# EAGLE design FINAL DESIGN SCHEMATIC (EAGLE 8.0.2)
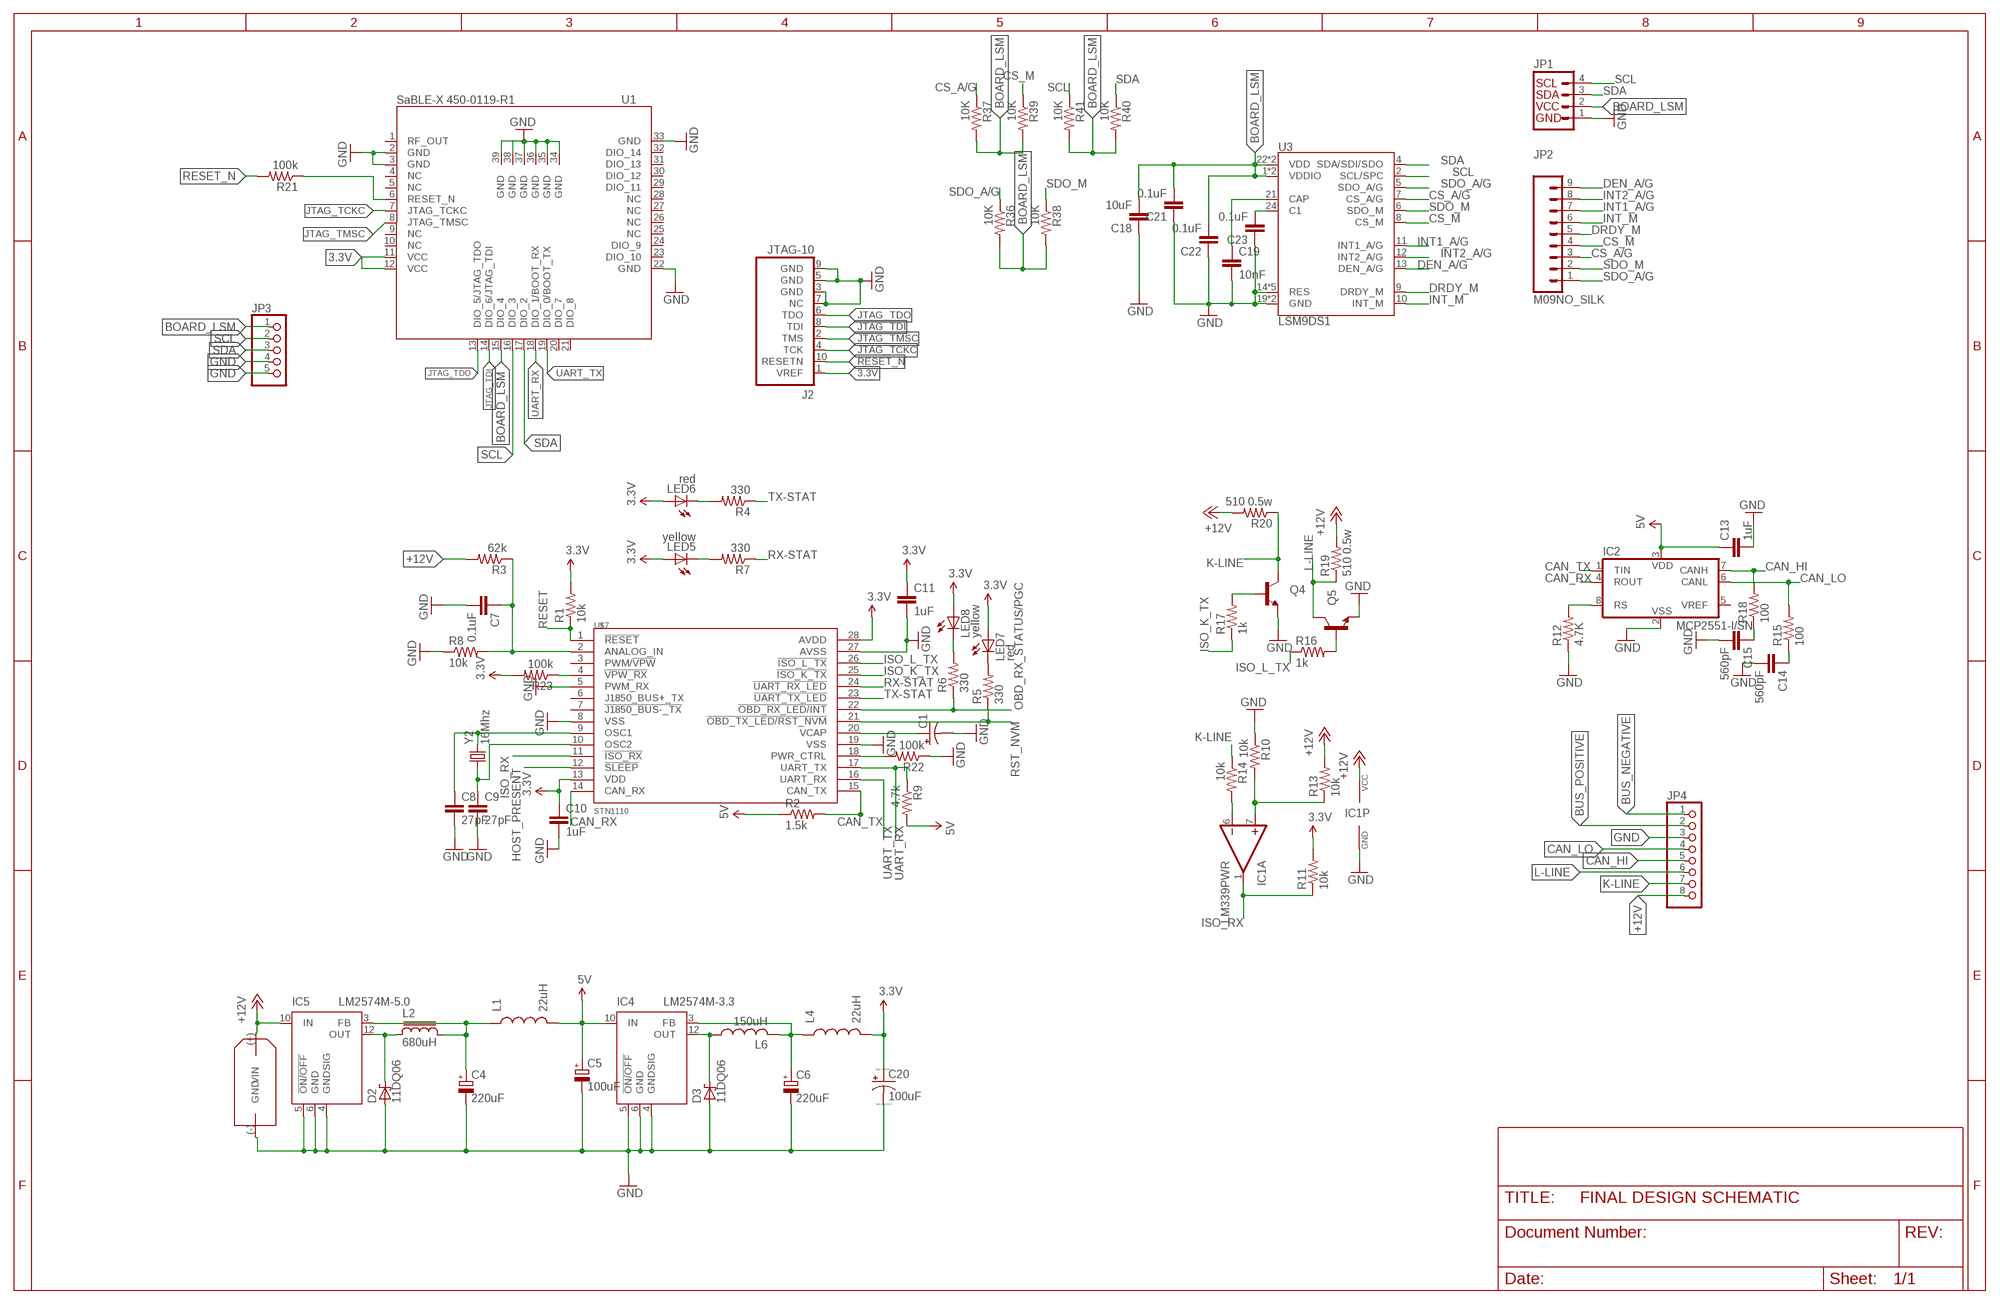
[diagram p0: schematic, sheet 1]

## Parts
C1  CAP_POL1206  [EIA3216]
C4  220uF  CPOL-EUUD-8X10  [UD-8X10_NICHICON]
C5  100uF  CPOL-EUUD-8X10  [UD-8X10_NICHICON]
C6  220uF  CPOL-EUUD-6,3X7,7  [UD-6,3X7,7_NICHICON]
C7  0.1uF  CAP0402-CAP  [0402-CAP]
C8  27pF  CAP0402-CAP  [0402-CAP]
C9  27pF  CAP0402-CAP  [0402-CAP]
C10  1uF  CAP0402-CAP  [0402-CAP]
C11  1uF  CAP0402-CAP  [0402-CAP]
C13  1uF  CAP0402-CAP  [0402-CAP]
C14  560pF  CAP0402-CAP  [0402-CAP]
C15  560pF  CAP0402-CAP  [0402-CAP]
C18  10uF  10UF-6.3V-20%(0603)  [0603-CAP]
C19  10nF  10UF-6.3V-20%(0603)  [0603-CAP]
C20  100uF  CPOL-US139CLL-3R  [139CLL-3R]
C21  0.1uF  0.1UF-25V(+80/-20%)(0603)  [0603-CAP]
C22  0.1uF  0.1UF-25V(+80/-20%)(0603)  [0603-CAP]
C23  0.1uF  0.1UF-25V(+80/-20%)(0603)  [0603-CAP]
CIN1  22uF  MAL214699801E3  [146CTI]
D2  11DQ06  1N5817-T  [DO41-7.6]
D3  11DQ06  1N5817-T  [DO41-7.6]
IC1  LM339PWR  [TSSOP-14]
IC2  MCP2551-I/SN  [SO-8]
IC4  LM2574M-3.3  [SO14W]
IC5  LM2574M-5.0  [SO14W]
J2  JTAG-10  [JTAG-10]
JP1  I2C_STANDARD_NO_SILK  [1X04_NO_SILK]
JP2  M09NO_SILK  [1X09_NO_SILK]
JP3  PINHD-1X5  [1X05]
JP4  PINHD-1X8  [1X08]
L1  22uH  INDUCTOR1210  [1210]
L2  680uH  SDR1006  [SDR1006]
L4  22uH  INDUCTOR1210  [1210]
L6  150uH  L-USL1812  [L1812]
LED5  yellow  LED0603  [LED-0603]
LED6  red  LED0603  [LED-0603]
LED7  red  LED0603  [LED-0603]
LED8  yellow  LED0603  [LED-0603]
Q4  TRANSISTOR_NPNSOT23-3  [SOT23-3]
Q5  TRANSISTOR_NPNSOT23-3  [SOT23-3]
R1  10k  RESISTOR0402-RES  [0402-RES]
R2  1.5k  RESISTOR0402-RES  [0402-RES]
R3  62k  RESISTOR0402-RES  [0402-RES]
R4  330  RESISTOR0402-RES  [0402-RES]
R5  330  RESISTOR0402-RES  [0402-RES]
R6  330  RESISTOR0402-RES  [0402-RES]
R7  330  RESISTOR0402-RES  [0402-RES]
R8  10k  RESISTOR0402-RES  [0402-RES]
R9  4.7k  RESISTOR0402-RES  [0402-RES]
R10  10k  RESISTOR0402-RES  [0402-RES]
R11  10k  RESISTOR0402-RES  [0402-RES]
R12  4.7K  RESISTOR0402-RES  [0402-RES]
R13  10k  RESISTOR0402-RES  [0402-RES]
R14  10k  RESISTOR0402-RES  [0402-RES]
R15  100  RESISTOR0402-RES  [0402-RES]
R16  1k  RESISTOR0402-RES  [0402-RES]
R17  1k  RESISTOR0402-RES  [0402-RES]
R18  100  RESISTOR0402-RES  [0402-RES]
R19  510 0.5w  RESISTOR2010  [R2010]
R20  510 0.5w  RESISTOR2010  [R2010]
R21  100k  RESISTOR0402-RES  [0402-RES]
R22  100k  RESISTOR0402-RES  [0402-RES]
R23  100k  RESISTOR0402-RES  [0402-RES]
R36  10K  10KOHM-1/10W-1%(0603)0603  [0603-RES]
R37  10K  10KOHM-1/10W-1%(0603)0603  [0603-RES]
R38  10K  10KOHM-1/10W-1%(0603)0603  [0603-RES]
R39  10K  10KOHM-1/10W-1%(0603)0603  [0603-RES]
R40  10K  10KOHM-1/10W-1%(0603)0603  [0603-RES]
R41  10K  10KOHM-1/10W-1%(0603)0603  [0603-RES]
U1  SABLEXTRACE-ANTENNA  [SABLEX_450-0119]
U3  LSM9DS1  [LGA24-8X4]
U$7  STN1110  [SO-28W]
Y2  16Mhz  CRYSTAL5X3  [CRYSTAL-SMD-5X3]

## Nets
3.3V [power]: C10.1 C11.1 C20.+ J2.1(VREF) L4.2 LED5.A LED6.A LED7.A LED8.A R1.2 R11.2 R23.2 U1.11(VCC) U1.12(VCC) U$7.13(VDD) U$7.28(AVDD)
5V [power]: C5.+ C13.1 IC2.3(VDD) IC4.10(IN) L1.2 R2.1 R9.2
+12V [power]: CIN1.(+)(VIN) IC1.3(P:VCC) IC5.10(IN) JP4.8 R3.2 R13.2 R19.2 R20.2
BOARD_LSM: C18.2 C21.2 C22.2 JP1.2 JP3.1 R36.2 R37.2 R38.2 R39.2 R40.2 R41.2 U1.15(DIO_4) U3.1(VDDIO) U3.3(VDDIO) U3.22(VDD) U3.23(VDD)
BUS_NEGATIVE: JP4.1
BUS_POSITIVE: JP4.2
CAN_HI: IC2.7(CANH) JP4.5 R18.2
CAN_LO: IC2.6(CANL) JP4.4 R15.2
CAN_RX: IC2.4(ROUT) U$7.14(CAN_RX)
CAN_TX: IC2.1(TIN) R2.2 U$7.15(CAN_TX)
CS_A/G: JP2.3 R37.1 U3.7(CS_A/G)
CS_M: JP2.4 R39.1 U3.8(CS_M)
DEN_A/G: JP2.9 U3.13(DEN_A/G)
DRDY_M: JP2.5 U3.9(DRDY_M)
GND [power]: C1.C(-) C4.- C5.- C6.- C7.2 C8.2 C9.2 C10.2 C11.2 C13.2 C14.2 C15.2 C18.1 C19.2 C20.- C21.1 C22.1 C23.1 CIN1.(-)(GND) D2.A D3.A IC1.12(P:GND) IC2.2(VSS) IC4.4(GNDSIG) IC4.5(!ON/OFF) IC4.6(GND) IC5.4(GNDSIG) IC5.5(!ON/OFF) IC5.6(GND) J2.3(GND) J2.5(GND) J2.7(NC) J2.9(GND) JP1.1 JP3.4 JP3.5 JP4.3 Q4.2(E) Q5.2(E) R8.1 R10.1 R12.1 R22.1 U1.2(GND) U1.3(GND) U1.22(GND) U1.33(GND) U1.34(GND) U1.35(GND) U1.36(GND) U1.37(GND) U1.38(GND) U1.39(GND) U3.14(RES) U3.15(RES) U3.16(RES) U3.17(RES) U3.18(RES) U3.19(GND) U3.20(GND) U$7.5(PWM_RX) U$7.8(VSS) U$7.19(VSS) U$7.27(AVSS)
HOST_PRESENT: U$7.12(!SLEEP)
INT1_A/G: JP2.7 U3.11(INT1_A/G)
INT2_A/G: JP2.8 U3.12(INT2_A/G)
INT_M: JP2.6 U3.10(INT_M)
ISO_K_TX: R17.1 U$7.25(!ISO_K_TX)
ISO_L_TX: R16.1 U$7.26(!ISO_L_TX)
ISO_RX: IC1.1(A:OUT) R11.1 U$7.11(!ISO_RX)
JTAG_TCKC: J2.4(TCK) U1.7(JTAG_TCKC)
JTAG_TDI: J2.8(TDI) U1.14(DIO_6/JTAG_TDI)
JTAG_TDO: J2.6(TDO) U1.13(DIO_5/JTAG_TDO)
JTAG_TMSC: J2.2(TMS) U1.8(JTAG_TMSC)
K-LINE: JP4.7 Q4.3(C) R14.1 R20.1
L-LINE: JP4.6 Q5.3(C) R19.1
N$1 [power]: C8.1 U$7.9(OSC1) Y2.3
N$2: R23.1 U$7.4(!VPW_RX)
N$3 [power]: D3.C IC4.12(OUT) L6.1
N$4 [power]: C4.+ IC5.3(FB) L1.1 L2.2
N$5 [power]: D2.C IC5.12(OUT) L2.1
N$6: R21.1 U1.6(RESET_N)
N$7: R22.2 U$7.18(PWR_CTRL)
N$8 [power]: C6.+ IC4.3(FB) L4.1 L6.2
N$11: LED7.C R5.2
N$15: C19.1 U3.21(CAP)
N$16: C23.2 U3.24(C1)
N$29: Q4.1(B) R17.2
N$34: IC2.8(RS) R12.2
N$35: IC1.7(A:+IN) R10.2 R13.1
N$40: C15.1 R18.1
N$41: C14.1 R15.1
N$42: IC1.6(A:-IN) R14.2
N$43: Q5.1(B) R16.2
N$44: C9.1 U$7.10(OSC2) Y2.1
N$47: C7.1 R3.1 R8.2 U$7.2(ANALOG_IN)
N$48: LED5.C R7.2
N$49: C1.A(+) U$7.20(VCAP)
N$50: LED8.C R6.2
N$51: LED6.C R4.2
OBD_RX_STATUS/PGC: R6.1 U$7.22(!OBD_RX_LED/INT)
RESET: R1.1 U$7.1(!RESET)
RESET_N: J2.10(RESETN) R21.2
RST_NVM: R5.1 U$7.21(!OBD_TX_LED/RST_NVM)
RX-STAT: R7.1 U$7.24(!UART_RX_LED)
SCL: JP1.4 JP3.2 R41.1 U1.16(DIO_3) U3.2(SCL/SPC)
SDA: JP1.3 JP3.3 R40.1 U1.17(DIO_2) U3.4(SDA/SDI/SDO)
SDO_A/G: JP2.1 R36.1 U3.5(SDO_A/G)
SDO_M: JP2.2 R38.1 U3.6(SDO_M)
TX-STAT: R4.1 U$7.23(!UART_TX_LED)
UART_RX: R9.1 U1.18(DIO_1/BOOT_RX) U$7.17(UART_TX)
UART_TX: U1.19(DIO_0/BOOT_TX) U$7.16(UART_RX)
Unconnected: IC1.2(B:OUT) IC1.4(B:-IN) IC1.5(B:+IN) IC1.8(C:-IN) IC1.9(C:+IN) IC1.10(D:-IN) IC1.11(D:+IN) IC1.13(D:OUT) IC1.14(C:OUT) IC2.5(VREF) U1.1(RF_OUT) U1.4(NC) U1.5(NC) U1.9(NC) U1.10(NC) U1.20(DIO_7) U1.21(DIO_8) U1.23(DIO_10) U1.24(DIO_9) U1.25(NC) U1.26(NC) U1.27(NC) U1.28(NC) U1.29(DIO_11) U1.30(DIO_12) U1.31(DIO_13) U1.32(DIO_14) U$7.3(PWM/!VPW) U$7.6(J1850_BUS+_TX) U$7.7(!J1850_BUS-_TX)

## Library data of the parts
C1 = OBD-II-UART-v13:CAP_POL: Capacitor Polarized
C4-C6 = FINAL DESIGN SCHEMATIC (Updated):CPOL-EU: POLARIZED CAPACITOR, European symbol
C7-C11 C13 = OBD-II-UART-v13:CAP: Capacitor; MPN: 2450L/C402D; OC_NEWARK: 55T4197
C14 C15 = OBD-II-UART-v13:CAP: Capacitor; OC_NEWARK: unknown
C18 = SparkFun-LSM9DS1-Breakout:10UF-6.3V-20%(0603): CAP-11015; OC_NEWARK: unknown; PROD_ID: CAP-11015
C19 = SparkFun-LSM9DS1-Breakout:10UF-6.3V-20%(0603): CAP-11015; OC_NEWARK: unknown; PROD_ID: CAP-11015; VALUE: 10uF
C20 = resistor:CPOL-US: POLARIZED CAPACITOR, American symbol
C21-C23 = SparkFun-LSM9DS1-Breakout:0.1UF-25V(+80/-20%)(0603): CAP-00810; OC_NEWARK: unknown; PROD_ID: CAP-00810
CIN1 = FINAL DESIGN SCHEMATIC (Updated):MAL214699801E3
D2 D3 = diode:1N581*: 1.0A SCHOTTKY BARRIER RECTIFIER
IC1 = OBD-II-UART-v13:LM339PWR: Quad Differential Comparators Based on information from the SLCS006N datasheet from TI (www.ti.com). Change Log DateAuthorChange July 16, 2008nick@scantool.netDevice created.; DESC: IC, Quad Comparator; MANUF: Texas Instruments; OC_NEWARK: unknown; PARTNUM: LM339PWR; SUPPLIER: Digikey:296-6607-1-ND; VALSTAT: PARTNUM
IC2 = OBD-II-UART-v13:MCP2551: CAN Driver Based on information from the MPC2551 datasheet from Microchip. http://www.microchip.com/ Change Log DateAuthorChange November 12, 2008joe@scantool.netRenamed "TXD" to "TIN" and "RXD" to "ROUT" Fixed mislabeled pins "CANH" and CANL"; DESC: IC, CAN Transceiver; MANUF: Microchip Technology; OC_NEWARK: unknown; PARTNUM: MCP2551-I/SN; SUPPLIER: Digikey:MCP2551-I/SN-ND; VALSTAT: PARTNUM
IC4 IC5 = linear:LM2574?-*: SIMPLE SWITCHER 0.5A Step-Down Voltage Regulator Source: http://cache.national.com/ds/LM/LM2574.pdf
J2 = luminary-arm:JTAG-10: JTAG 10-Pin Programming/Debug Connector
JP1 = SparkFun-LSM9DS1-Breakout:I2C_STANDARD: SparkFun has standardized on a pinout for all I2C based sensor breakouts. This pinout allows I2C boards to be plugged directly into the headers on Arduino Uno compatible boards, and to be daisy chained easily.; OC_NEWARK: unknown
JP2 = SparkFun-LSM9DS1-Breakout:M09: Header 9 Standard 9-pin 0.1" header. Use with straight break away headers (SKU : PRT-00116), right angle break away headers (PRT-00553), swiss pins (PRT-00743), machine pins (PRT-00117), and female headers (PRT-00115).; OC_NEWARK: unknown
JP3 = pinhead:PINHD-1X5: PIN HEADER
JP4 = pinhead:PINHD-1X8: PIN HEADER
L1 L4 = SparkFun-Passives:INDUCTOR: Inductors
L2 = inductor-bourns:SDR1006: POWER INDUCTOR
L6 = resistor:L-US: INDUCTOR, American symbol
LED5-LED8 = OBD-II-UART-v13:LED: LEDs; OC_NEWARK: unknown
Q4 Q5 = OBD-II-UART-v13:TRANSISTOR_NPN: Transistor NPN BJT configuration in SOT23 package. MMBT2222 is the common NPN we use. Double check BCE configuration again layout.; OC_NEWARK: unknown
R1-R23 = OBD-II-UART-v13:RESISTOR: Resistor; OC_NEWARK: unknown
R36-R41 = SparkFun-LSM9DS1-Breakout:10KOHM-1/10W-1%(0603): RES-00824; OC_NEWARK: unknown; PROD_ID: RES-00824
U1 = sablex:SABLEX: LSR SaBLE-x 450-0119-R1 Technical Specifications: Product Description: Bluetooth Low Energy Wireless Module VCC: 1.8v - 3.8v Operating Temperature: -40c - 85c Weight: 0.75g +/- 0.05f; OC_NEWARK: unknown
U3 = SparkFun-LSM9DS1-Breakout:LSM9DS1: LSM9DS1 3D accelerometer, gyroscope & magnetometer The LSM9DS1 is a system-in-package featuring a 3D digital linear acceleration sensor, a 3D digital angular rate sensor, and a 3D digital magnetic sensor. The LSM9DS1 has a linear acceleration full scale of ±2g/±4g/±8/±16 g, a magnetic field full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; OC_NEWARK: unknown; PROD_ID: IC-12536
U$7 = obd:STN1110: Multiprotocol OBD to UART Interpreter; OC_NEWARK: unknown
Y2 = OBD-II-UART-v13:CRYSTAL: Crystals; OC_NEWARK: unknown

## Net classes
0 default_signal: width 0.01 mm
1 power: width 0.015 mm

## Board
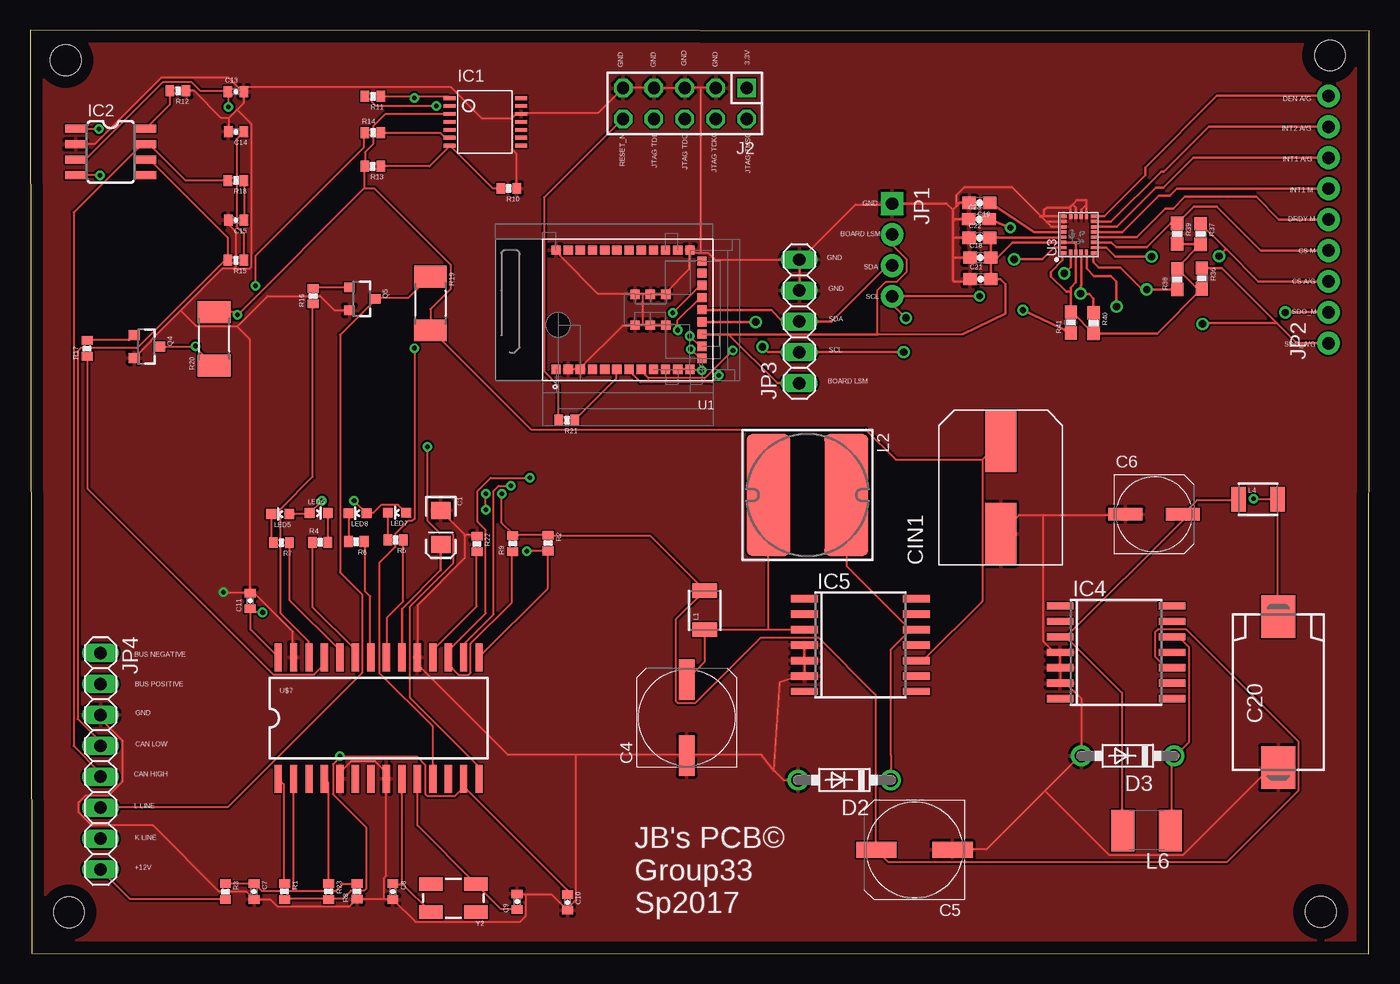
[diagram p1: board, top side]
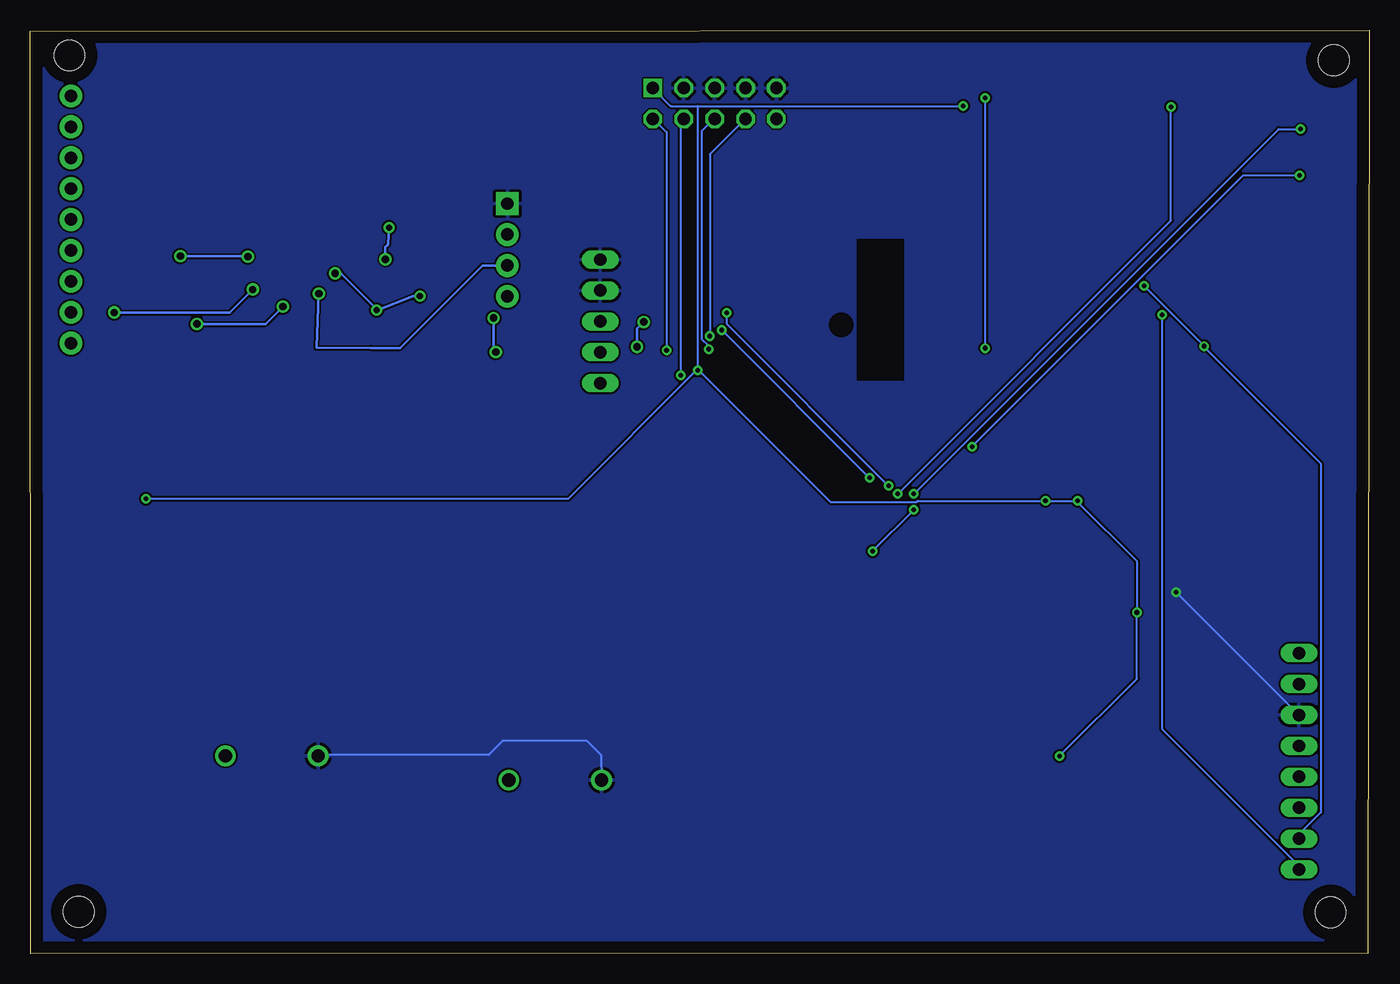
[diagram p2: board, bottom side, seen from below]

Size 109.96 x 75.84 mm. Coordinates in mm from the lower left corner, seen from the top.
Outline: 0.09,0.04 109.94,0 109.96,75.76 0,75.84 0.09,0.04
Copper layers (1*16): Top 0.035mm / dielectric 1.5mm / Bottom 0.035mm
Design rules "default *": minimum track width 7mil, minimum drill 15mil, track to track 6mil, track to pad 6mil, pad to pad 6mil, via to via 6mil, smd to smd 6mil, copper to edge 40mil, drill to drill 8mil, minimum pad ring 10mil, minimum via ring 8mil, stop-mask expansion 4mil, vias tented up to drill 0mil, thermal gap 10mil
Holes 2.5 mm at 2.9,73.4 3.15,3.39 105.98,3.43 106.74,73.79

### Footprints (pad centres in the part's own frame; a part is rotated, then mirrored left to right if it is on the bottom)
EIA3216 = smd 1.4 x 1.6: A 1.4,0; C -1.4,0
UD-8X10_NICHICON = smd 3.3 x 1.3: + 3.125,0; - -3.125,0
UD-6,3X7,7_NICHICON = smd 2.8 x 1: + 2.35,0; - -2.35,0
0402-CAP = smd 0.7 x 0.9: 1 -0.65,0; 2 0.65,0
0603-CAP = smd 1.1 x 1: 1 -0.85,0; 2 0.85,0
139CLL-3R = smd 3.5 x 2.8: + 6.2,0; - -6.2,0
146CTI = smd 5.08 x 2.54: (+) 10.16,0; (-) 2.54,0
DO41-7.6 = drill 1.1 pad 1.7: A 3.81,0; C -3.81,0
TSSOP-14 = smd 0.305 x 0.991: 1 -1.95,-2.925; 2 -1.3,-2.925; 3 -0.65,-2.925; 4 0,-2.925; 5 0.65,-2.925; 6 1.3,-2.925; 7 1.95,-2.925; 8 1.95,2.925; 9 1.3,2.925; 10 0.65,2.925; 11 0,2.925; 12 -0.65,2.925; 13 -1.3,2.925; 14 -1.95,2.925
SO-8 = smd 0.65 x 1.75: 1 -1.905,-2.873; 2 -0.635,-2.873; 3 0.635,-2.873; 4 1.905,-2.873; 5 1.905,2.873; 6 0.635,2.873; 7 -0.635,2.873; 8 -1.905,2.873
SO14W = smd 0.6 x 2.2: 1 -3.81,-4.6; 2 -2.54,-4.6; 3 -1.27,-4.6; 4 0,-4.6; 5 1.27,-4.6; 6 2.54,-4.6; 7 3.81,-4.6; 8 3.81,4.6; 9 2.54,4.6; 10 1.27,4.6; 11 0,4.6; 12 -1.27,4.6; 13 -2.54,4.6; 14 -3.81,4.6
JTAG-10 = drill 1.016 square: 1 -5.08,-1.27 | drill 1.016 octagon: 2 -5.08,1.27; 3 -2.54,-1.27; 4 -2.54,1.27; 5 0,-1.27; 6 0,1.27; 7 2.54,-1.27; 8 2.54,1.27; 9 5.08,-1.27; 10 5.08,1.27
1X04_NO_SILK = drill 1.016 pad 1.88 square: 1 0,0 | drill 1.016 pad 1.88: 2 2.54,0; 3 5.08,0; 4 7.62,0
1X09_NO_SILK = drill 1.016 pad 1.88: 1 0,0; 2 2.54,0; 3 5.08,0; 4 7.62,0; 5 10.16,0; 6 12.7,0; 7 15.24,0; 8 17.78,0; 9 20.32,0
1X05 = drill 1.016 long: 1 -5.08,0; 2 -2.54,0; 3 0,0; 4 2.54,0; 5 5.08,0
1X08 = drill 1.016 long: 1 -8.89,0; 2 -6.35,0; 3 -3.81,0; 4 -1.27,0; 5 1.27,0; 6 3.81,0; 7 6.35,0; 8 8.89,0
1210 = smd 1.2 x 2: 1 -1.6,0; 2 1.6,0
SDR1006 = smd 10 x 3.6: 1 0,3.2; 2 0,-3.2
L1812 = smd 1.9 x 3.4: 1 -1.95,0; 2 1.95,0
LED-0603 = smd 0.8 x 0.8: A 0,-0.75; C 0,0.75
SOT23-3 = smd 0.8 x 0.9: 1 -0.95,-1; 2 0.95,-1; 3 0,1.1
0402-RES = smd 0.7 x 0.9: 1 -0.65,0; 2 0.65,0
R2010 = smd 1.8 x 2.7: 1 -2.2,0; 2 2.2,0
0603-RES = smd 1.1 x 1: 1 -0.85,0; 2 0.85,0
SABLEX_450-0119 = smd 0.76 x 0.76: 1 -4.905,5.91; 2 -4.905,4.91; 3 -4.905,3.91; 4 -4.905,2.91; 5 -4.905,1.91; 6 -4.905,0.91; 7 -4.905,-0.09; 8 -4.905,-1.09; 9 -4.905,-2.09; 10 -4.905,-3.09; 11 -4.905,-4.09; 12 -4.905,-5.09; 13 -4,-6.09; 14 -3,-6.09; 15 -2,-6.09; 16 -1,-6.09; 17 0,-6.09; 18 1,-6.09; 19 2,-6.09; 20 3,-6.09; 21 4,-6.09; 22 4.905,-5.09; 23 4.905,-4.09; 24 4.905,-3.09; 25 4.905,-2.09; 26 4.905,-1.09; 27 4.905,-0.09; 28 4.905,0.91; 29 4.905,1.91; 30 4.905,2.91; 31 4.905,3.91; 32 4.905,4.91; 33 4.905,5.91; 34 -1.27,-0.57; 35 -1.27,-1.84; 36 -1.27,-3.11; 37 1.27,-0.57; 38 1.27,-1.84; 39 1.27,-3.11
LGA24-8X4 = smd 0.27 x 0.45: 1 -1.505,1.225; 6 -1.505,-1.225; 7 -1.075,-1.225; 8 -0.645,-1.225; 9 -0.215,-1.225; 10 0.215,-1.225; 11 0.645,-1.225; 12 1.075,-1.225; 13 1.505,-1.225; 18 1.505,1.225; 19 1.075,1.225; 20 0.645,1.225; 21 0.215,1.225; 22 -0.215,1.225; 23 -0.645,1.225; 24 -1.075,1.225 | smd 0.45 x 0.27: 2 -1.475,0.645; 3 -1.475,0.215; 4 -1.475,-0.215; 5 -1.475,-0.645; 14 1.475,-0.645; 15 1.475,-0.215; 16 1.475,0.215; 17 1.475,0.645
SO-28W = smd 0.6 x 2.3: 1 -8.255,-5; 2 -6.985,-5; 3 -5.715,-5; 4 -4.445,-5; 5 -3.175,-5; 6 -1.905,-5; 7 -0.635,-5; 8 0.635,-5; 9 1.905,-5; 10 3.175,-5; 11 4.445,-5; 12 5.715,-5; 13 6.985,-5; 14 8.255,-5; 15 8.255,5; 16 6.985,5; 17 5.715,5; 18 4.445,5; 19 3.175,5; 20 1.905,5; 21 0.635,5; 22 -0.635,5; 23 -1.905,5; 24 -3.175,5; 25 -4.445,5; 26 -5.715,5; 27 -6.985,5; 28 -8.255,5
CRYSTAL-SMD-5X3 = smd 1.9 x 1.1: 1 -1.85,-1.15; 2 1.85,-1.15; 3 1.85,1.15; 4 -1.85,1.15

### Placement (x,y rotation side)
C1  33.71,34.99 270 top
C4  53.91,19.38 90 top
C5  72.62,8.51 180 top
C6  92.3,36.09 0 top
C7  18.36,5.1 270 top
C8  29.77,5.09 270 top
C9  39.99,4.26 90 top
C10  44.12,4.21 270 top
C11  18.05,28.97 90 top
C13  16.87,70.81 0 top
C14  16.9,67.5 180 top
C15  16.9,60.24 180 top
C18  78.02,57.17 0 top
C19  77.96,61.67 180 top
C20  102.5,21.47 90 top
C21  78.04,55.41 0 top
C22  77.95,58.8 0 top
C23  77.91,60.32 0 top
CIN1  79.71,31.94 90 top
D2  66.86,14.25 180 top
D3  90.14,16.24 180 top
IC1  37.36,68.32 270 top
IC2  6.6,65.85 270 top
IC4  89.17,24.75 270 top
IC5  68.18,25.34 270 top
J2  53.76,69.84 180 top
JP1  70.78,61.61 270 top
JP2  106.63,50.14 90 top
JP3  63.15,51.93 90 top
JP4  5.76,15.79 270 top
L1  55.39,28.2 90 top
L2  63.82,37.67 270 top
L4  100.84,37.33 0 top
L6  91.68,10.11 180 top
LED5  20.53,36.1 90 top
LED6  23.69,36.19 270 top
LED7  30.11,36.21 90 top
LED8  26.86,36.17 90 top
Q4  9.51,49.87 270 top
Q5  27.2,53.79 270 top
R1  20.86,5.1 270 top
R2  42.52,33.72 270 top
R3  16.02,5.08 270 top
R4  23.8,33.78 0 top
R5  29.99,33.98 180 top
R6  26.76,33.84 180 top
R7  20.62,33.75 180 top
R8  26.82,5.12 90 top
R9  39.62,33.67 90 top
R10  39.29,62.86 180 top
R11  28.13,70.43 180 top
R12  12.13,70.87 180 top
R13  28.12,64.68 180 top
R14  28.13,67.44 0 top
R15  16.88,56.95 180 top
R16  23.22,54.02 90 top
R17  4.65,49.71 90 top
R18  16.89,63.5 180 top
R19  32.84,53.4 270 top
R20  15.09,50.5 90 top
R21  44.06,43.82 180 top
R22  36.67,33.65 270 top
R23  24.49,5.1 270 top
R36  96.22,55.46 270 top
R37  96.11,59.11 270 top
R38  94.2,55.41 90 top
R39  94.19,59.14 270 top
R40  87.33,51.8 270 top
R41  85.46,51.85 90 top
U1  49.08,52.89 90 top
U3  86.09,59.07 90 top
U$7  28.6,19.34 0 top
Y2  34.74,4.56 180 top

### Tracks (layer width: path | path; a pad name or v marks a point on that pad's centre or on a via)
3.3V  (via drill 0.38)
  Top 0.178: U$7.28 20.31,24.39 18.08,26.62 18.08,28.27 C11.1 18.16,28.03 v19.07,28.03 | LED5.A 21.3,36.12 22.87,36.12 LED6.A 22.95,36.2 v23.94,37.19 | LED7.A 30.79,36.28 30.22,36.86 28.81,36.86 28.15,36.2 27.66,36.2 LED8.A 27.57,36.2 v26.58,37.19 | R1.2 20.89,4.5 24.44,4.5 R23.2 24.52,4.5 25.67,4.5 26.34,5.16 27.41,5.16 27.57,5.33 27.57,10.36 24.85,13.09 24.85,15.56 25.43,16.14 | C10.1 44.08,4.91 44.08,5.24 35.66,13.66 35.66,14.32 U$7.13 35.58,13.66 34.84,12.92 32.61,12.92 32.44,13.09 32.44,15.48 31.78,16.14 25.43,16.14 | v25.43,16.22 25.43,16.14 | C20.+ 102.45,27.7 102.45,37.27 L4.2 102.36,37.36 v100.47,37.36 | U1.11 53.25,48 54.15,48 U1.12 54.24,47.92 v55.15,47.92 | v33.35,69.63 28.4,69.63 27.66,70.38 27.49,70.38 R11.2
  Bottom 0.178: v25.43,16.22 19.07,22.58 v19.07,28.03 19.07,32.24 23.94,37.11 v23.94,37.19 v26.58,37.19 37.07,37.19 37.15,37.11 44.25,37.11 55.06,47.92 v55.15,47.92 | 55.15,69.63 57.37,69.63 58.78,71.04 J2.1 | 55.15,69.63 v33.35,69.63 | 55.15,69.63 v55.15,47.92 | v100.47,37.36 65.79,37.36 55.23,47.92 v55.15,47.92
5V  (via drill 0.38)
  Top 0.178: IC4.10 93.7,23.49 93.28,23.49 92.38,24.39 92.38,26.38 92.62,26.62 94.93,26.62 104.18,17.38 104.18,13.42 98.32,7.55 70.42,7.55 69.51,8.46 C5.+ 69.43,8.55 69.43,21.26 64.72,25.96 60.02,25.96 54.65,20.6 53.16,20.6 53,20.76 53,27.45 55.31,29.76 L1.2 55.39,29.84 50.94,34.3 42.6,34.3 R2.1 42.52,34.38 39.63,34.38 R9.2 39.63,34.47 38.72,35.37 v38.72,37.77 | IC2.3 3.8,65.26 4.54,65.26 10.9,71.61 13.21,71.61 13.95,70.87 16.18,70.87 C13.1 16.26,70.79 v16.26,69.55
  Bottom 0.178: v16.26,69.55 16.26,60.22 v38.72,37.77
+12V  (via drill 0.38)
  Top 0.178: 78.18,40.57 78.18,28.93 73.39,24.15 72.81,24.15 IC5.10 | 78.18,40.57 79.66,42.06 CIN1.(+) | R3.2 15.93,4.5 8.17,4.5 5.78,6.89 JP4.8 | IC1.3 29.14,68.97 28.15,67.98 28.15,66.5 27.49,65.83 27.49,64.68 R13.2 27.41,64.6 27.41,62.86 | 17.01,52.71 17.25,52.71 27.41,62.86 | 17.01,52.71 15.11,52.71 R20.2 | 27.41,62.86 28.23,62.86 34.51,56.59 34.51,54.61 32.86,52.96 32.86,51.22 R19.2 32.94,51.22 41.11,43.05 68.6,43.05 71.08,40.57 78.18,40.57 | 17.01,52.71 v17.01,52.46
  Bottom 0.178: v17.01,52.46 17.01,18.45 5.78,7.22 5.78,6.98 JP4.8
BOARD_LSM
  Top 0.178: JP1.2 70.83,59.07 70.83,58.16 71.99,57 71.99,56.01 71.16,55.19 70.25,55.19 69.59,54.53 69.59,50.89 69.59,50.87
  Top 0.2: R41.2 | R41.2 85.57,52.7 R40.2 92.56,50.95 R36.2 95.84,54.61 R38.2 94.2,56.35 R37.2 94.22,58.26 R39.2 | R41.2 85.46,54.37 | 85.46,54.37 85.46,54.72 85.89,55.15 85.89,57.58 U3.3 85.86,57.61 85.86,58.42 85.85,58.42 U3.23 80.66,58.42 79.41,57.17 C18.2 | U3.1 | C18.2 78.89,57.16 C21.2 79.66,55.41 80.07,55 80.07,52.56 76.6,50.88 69.59,50.87 57.35,50.85 | C18.2 78.87,58.73 C22.2 84.82,58.8 U3.22 | 85.46,54.37 85.08,54.37 83.83,55.62 83.83,56 84.78,56.95 84.78,57.47 U3.1 | 57.35,50.85 55.22,50.84 U1.15 | JP3.1 61.35,46.85 57.35,50.85
CAN_HI
  Top 0.178: R18.2 16.18,63.52 12.71,63.52 9.83,66.41 9.5,66.41 IC2.7 9.41,66.41 9.08,66.41 3.55,60.88 3.55,17.05 5.7,14.9 5.7,14.57 JP4.5
CAN_LO
  Top 0.178: IC2.6 9.5,65.17 9.83,65.17 16.18,58.82 16.18,57 R15.2 16.1,57.08 8.75,49.74 4.13,49.74 3.88,49.49 3.88,19.28 5.7,17.46 5.7,17.13 JP4.4
CAN_RX  (via drill 0.38)
  Top 0.178: v5.7,63.94 3.8,63.94 IC2.4 | v32.61,41.65 32.61,35.54 33.6,34.55 34.59,34.55 34.76,34.38 34.76,32.07 31.21,28.52 31.21,21.01 36.82,15.4 36.82,14.41 U$7.14
  Bottom 0.178: v5.7,63.94 10.32,63.94 v32.61,41.65
CAN_TX  (via drill 0.38)
  Top 0.178: U$7.15 36.9,24.39 42.52,30.01 R2.2 42.43,33.06 v40.78,33.06 | v5.62,67.73 3.8,67.73 IC2.1 | v37.4,36.45 v37.4,37.77
  Bottom 0.178: v5.62,67.73 7.43,67.73 v37.4,37.77 | v40.78,33.06 v37.4,36.45
CS_A/G  (via drill 0.6)
  Top 0.2: JP2.3 100.86,55.22 98.26,57.81 | 98.26,57.81 R37.1 | 98.26,57.81 98.15,57.81 v97.64,57.29 | v92.1,57.25 89.1,57.25 88.36,57.99 U3.7
  Bottom 0.2: v97.64,57.29 92.14,57.29 v92.1,57.25
CS_M
  Top 0.2: JP2.4 101.08,57.76 97.47,61.37 95.57,61.37 R39.1 93.65,59.99 91.7,58.03 89.2,58.03 88.81,58.42 U3.8
DEN_A/G
  Top 0.2: JP2.9 97.46,70.46 91.58,64.57 91.58,63.94 88.22,60.58 87.33,60.58 U3.13
DRDY_M
  Top 0.2: JP2.5 102.55,60.3 100.69,62.16 94.83,62.16 93.88,61.21 93.22,61.21 90.87,58.86 87.33,58.86 U3.9
GND  (via drill 0.38)
  Top 0.178: 55.06,71.12 56.22,71.12 J2.3 | 55.06,71.12 53.82,71.12 J2.5 53.74,71.12 51.27,71.12 J2.7 51.18,71.12 48.71,71.12 J2.9 48.62,71.04 46.64,69.05 40.37,69.05 IC1.12 39.87,68.97 39.54,68.64 | 39.54,68.64 39.54,66.08 39.87,65.75 39.87,62.86 R10.1 | U1.2 44.25,48 45.16,48 U1.3 45.16,48.09 48.62,51.55 49.61,51.55 U1.34 49.7,51.64 50.27,51.64 | 50.27,51.64 50.85,51.64 U1.35 50.94,51.64 52.17,51.64 U1.36 | JP3.5 JP3.4 | 50.27,54.2 50.85,54.2 U1.38 50.94,54.2 52.17,54.2 U1.39 52.17,54.28 54.15,56.26 54.15,57.74 U1.22 54.24,57.58 55.06,57.58 | 50.27,54.2 49.7,54.2 U1.37 49.61,54.2 46.64,54.2 43.51,57.33 43.51,57.41 43.18,57.74 U1.33 | 55.06,57.58 55.64,57.58 56.22,57 63.07,57 JP3.5 | 50.27,54.2 50.27,51.64 | JP1.1 70.75,61.54 67.78,61.54 63.24,57 JP3.5 | 55.06,57.58 55.06,71.12 | 16.26,68.64 16.26,67.57 C14.2 | 16.97,69.34 17.5,69.88 17.5,70.79 C13.2 | 16.97,69.34 16.26,68.64 | 16.26,68.64 15.69,68.64 13.46,70.87 12.8,70.87 R12.1 | IC2.2 3.8,66.5 5.29,66.5 10.73,71.94 16.26,71.94 17.42,70.79 C13.2 | C11.2 18.08,29.6 18.41,29.6 21.55,26.46 21.55,24.39 U$7.27 | 12.34,52.83 15.77,56.26 16.68,56.26 | 12.34,52.83 9.91,50.4 9.91,50.32 8.59,48.99 Q4.2 | 16.68,56.26 16.84,56.42 16.84,59.31 16.26,59.89 16.26,60.22 C15.2 | 17.01,51.55 19.48,54.03 23.78,54.03 24.93,52.87 26.17,52.87 Q5.2 | 17.01,51.55 13.62,51.55 12.34,52.83 | C11.2 18,29.68 18,50.48 17.01,51.47 17.01,51.55 | 16.97,69.34 18.16,68.15 18.16,56.42 18,56.26 16.68,56.26 | 39.54,68.64 37.07,68.64 34.51,71.2 17.92,71.2 17.59,70.87 C13.2 | 83.21,36.03 81.23,36.03 79.75,34.55 CIN1.(-) | 83.21,36.03 89.9,36.03 C6.- | 83.34,13.37 86.27,16.3 D3.A 86.35,16.3 86.35,20.93 85.03,22.25 84.7,22.25 IC4.6 84.62,22.25 84.62,23.4 IC4.5 84.62,23.49 84.62,24.72 IC4.4 84.53,24.81 84.04,24.81 83.21,25.63 83.21,36.03
  Top 0.178: 83.34,13.37 78.51,8.55 75.78,8.55 C5.- | 83.34,13.37 88.58,8.13 94.69,8.13 101.79,15.23 102.45,15.23 C20.- | R22.1 36.65,34.38 35.77,34.38 35.66,34.38 35.66,32.48 31.78,28.6 31.78,24.39 U$7.19 31.78,24.31 31.78,23.73 39.21,16.3 44.83,16.3 | IC5.4 63.57,25.3 63.57,24.15 IC5.5 63.57,22.83 IC5.6 63.48,22.83 63.07,22.83 61.56,22.31 61.08,15.05 | 61.08,15.05 61.91,14.22 D2.A | 61.08,15.05 61.13,14.98 60.07,16.34 53.99,16.3 C4.- 53.91,16.3 44.83,16.3 | U$7.5 25.43,14.41 25.43,14.9 26.34,15.81 28.32,15.81 29.22,14.9 29.22,14.41 U$7.8 29.22,14.32 29.22,6.4 29.06,6.23 29.06,4.5 | 40.7,4.83 42.85,4.83 44.08,3.59 C10.2 44.08,3.67 44.83,4.42 44.83,16.3 | 40.7,4.83 40.04,4.83 C9.2 | 29.06,4.5 26.83,4.5 R8.1 26.75,4.42 26.17,3.84 20.31,3.84 19.73,4.42 18.41,4.42 C7.2 18.33,4.5 17.75,5.08 15.52,5.08 10.07,10.53 5.04,10.53 3.96,11.6 3.96,12.43 4.54,13 6.44,13 7.6,14.16 7.6,17.46 5.78,19.28 5.78,19.52 JP4.3 | 29.06,4.5 29.72,4.5 C8.2 29.8,4.42 31.62,2.6 40.2,2.6 40.7,3.1 40.7,4.83 | v15.85,29.68 17.92,29.68 C11.2
  Top 0.2: C19.2 76.32,61.67 76.05,61.41 | 76.05,61.41 75.76,61.11 | 75.76,58.68 75.76,57.14 | 75.76,60.14 75.76,58.68 | 75.76,60.14 75.76,61.11 | 75.76,57.14 75.76,55.31 75.86,55.21 76.99,55.21 C21.1 | C18.1 75.79,57.17 75.76,57.14 | C22.1 75.88,58.8 75.76,58.68 | C23.1 75.94,60.32 75.76,60.14 | 75.76,61.11 75.26,61.61 JP1.1 | 86.74,61.54 U3.14 | 86.74,61.54 86.74,61.9 86.73,61.9 85.97,61.9 85.62,61.54 | 85.62,61.54 85.44,61.37 | 85.44,61.37 U3.17 | U3.16 85.88,61.28 85.62,61.54 | U3.15 86.31,61.11 86.74,61.54 | U3.20 83.87,59.71 83.51,60.07 | 83.51,60.07 83.51,60.15 83.51,60.14 U3.19 | 83.51,60.07 83.03,60.55 | 83.03,60.55 82.97,60.55 82.99,60.57 83.25,60.57 | 83.25,60.57 U3.18 | 85.44,61.37 85.36,61.29 83.48,61.29 83.25,61.06 83.25,60.57 | 83.03,60.55 80.61,62.97 76.73,62.97 76.05,62.29 76.05,61.41 | 35.66,34.38 35.66,34.44 | 35.77,34.38 35.71,34.38 C1.C
  Bottom 0.178: D3.A 86.35,16.3 72.32,16.3 71.16,17.46 64.23,17.46 63.07,16.3 D2.A | v15.85,29.68 5.78,19.61 JP4.3
  pour Top: -0.99,77.01 111.77,77.01 111.77,-1.36 -1.15,-1.36 -1.15,75.77
  pour Bottom: -1.15,77.17 111.44,77.17 111.44,-1.94 -1.56,-1.94 -1.56,75.77
INT1_A/G
  Top 0.2: JP2.7 95.52,65.38 93.06,62.91 92.44,62.91 89.23,59.7 U3.11
INT2_A/G
  Top 0.2: JP2.8 96.78,67.92 93.12,64.25 92.89,64.25 88.77,60.13 U3.12
INT_M
  Top 0.2: JP2.6 94.15,62.84 93.6,62.28 92.69,62.28 89.69,59.28 U3.10
ISO_K_TX
  Top 0.178: R17.1 4.71,48.99 4.71,38.18 19.98,22.91 23.28,22.91 24.11,23.73 24.11,24.31 U$7.25
ISO_L_TX
  Top 0.178: R16.1 23.2,53.29 23.2,39.17 20.56,36.53 20.56,27.94 22.87,25.63 22.87,24.39 U$7.26
ISO_RX  (via drill 0.38)
  Top 0.178: 31.54,70.38 34.34,70.38 34.43,70.29 IC1.1 | 31.54,70.38 28.81,70.38 R11.1 | v31.54,49.74 31.54,35.7 31.37,35.54 31.04,35.54 29.97,34.47 29.97,33.39 28.65,32.07 28.65,23.07 33.02,18.7 33.02,14.41 U$7.11 | v31.54,70.29 31.54,70.38
  Bottom 0.178: v31.54,70.29 v31.54,49.74
JTAG_TCKC  (via drill 0.38)
  Top 0.178: v56.55,47.51 55.97,46.93 50.11,46.93 49.53,47.51 49.53,47.59 49.2,47.92 U1.7
  Bottom 0.178: v56.55,47.51 56.55,68.31 56.3,68.56 J2.4
JTAG_TDI  (via drill 0.38)
  Top 0.178: v54.15,50.73 54.98,49.9 55.15,49.9 U1.14
  Bottom 0.178: v54.15,50.73 54.15,65.67 51.27,68.56 J2.8
JTAG_TDO  (via drill 0.38)
  Top 0.178: v54.24,49.66 54.98,48.91 55.15,48.91 U1.13
  Bottom 0.178: v54.24,49.66 54.24,49.9 54.82,50.48 54.82,67.57 53.82,68.56 J2.6
JTAG_TMSC  (via drill 0.38)
  Top 0.178: v57.7,49.57 55.39,47.26 50.77,47.26 50.52,47.51 50.52,47.59 50.19,47.92 U1.8
  Bottom 0.178: v57.7,49.57 57.7,67.49 58.78,68.56 J2.2
K-LINE  (via drill 0.38)
  Top 0.178: 13.54,49.82 10.65,49.82 Q4.3 | 13.54,49.82 15.03,48.33 R20.1 | v18.49,54.86 18.49,57.33 27.41,66.25 27.41,67.4 R14.1 | v13.54,49.9 13.54,49.82
  Bottom 0.178: v18.49,54.86 v13.54,49.9 13.54,49.82 3.96,40.24 3.96,11.6 5.7,9.87 5.7,9.45 JP4.7
L-LINE
  Top 0.178: R19.1 32.77,55.6 31.04,53.87 28.32,53.87 Q5.3 28.32,53.7 25.43,50.81 25.43,31.33 27.24,29.51 27.24,23.07 16.18,12.01 5.78,12.01 JP4.6
N$1
  Top 0.178: 30.55,5.66 30.63,5.66 32.86,3.43 Y2.3 | 30.55,5.66 29.8,5.66 C8.1 | 30.55,5.66 30.55,14.32 U$7.9
N$2
  Top 0.178: R23.1 24.44,5.82 24.44,14.08 24.19,14.32 U$7.4
N$3
  Top 0.178: IC4.12 93.78,25.96 94.36,25.96 95.18,25.14 95.18,17.38 94.11,16.3 D3.C 94.03,16.22 93.7,15.89 93.7,10.11 L6.1
N$4
  Top 0.178: C4.+ 53.99,22.58 55.39,23.98 55.39,26.54 L1.1 55.48,26.62 60.59,26.62 | 60.59,26.62 IC5.3 | 60.59,26.62 60.59,37.6 L2.2
N$5
  Top 0.178: D2.C 70.66,16.3 70.66,24.97 72.23,26.54 72.73,26.54 IC5.12 72.23,26.62 67.03,31.82 67.03,37.6 L2.1
N$6
  Top 0.178: U1.6 48.13,47.92 48.13,47.26 44.74,43.88 R21.1
N$7
  Top 0.178: R22.2 36.65,32.98 36.65,28.52 33.1,24.97 33.1,24.39 U$7.18
N$8
  Top 0.178: L4.1 99.23,37.27 95.84,37.27 94.69,36.12 C6.+ 94.6,36.03 94.6,35.54 85.11,26.05 84.62,26.05 IC4.3 85.11,25.96 89.65,21.42 89.65,10.11 L6.2
N$11
  Top 0.178: LED7.C 29.39,36.2 29.39,34.05 R5.2
N$15
  Top 0.2: C19.1 82.46,59.28 U3.21
N$16  (via drill 0.5, 0.6)
  Top 0.2: C23.2 80.06,59.79 v80.49,59.63 | U3.24 84.08,57.99 83.12,57.03 v80.8,57.03
  Bottom 0.2: v80.49,59.63 80.57,58.3 80.63,58.21 80.81,58.03 v80.8,57.03
N$29
  Top 0.178: R17.2 4.71,50.4 8.09,50.4 8.5,50.81 Q4.1
N$34
  Top 0.178: R12.2 11.48,69.8 9.5,67.82 IC2.8
N$35
  Top 0.178: R10.2 37.97,62.86 34.51,66.33 IC1.7 34.43,66.33 32.77,64.68 28.81,64.68 R13.1
N$40
  Top 0.178: R18.1 17.59,63.44 17.59,60.3 C15.1
N$41
  Top 0.178: R15.1 17.5,57 17.5,59.15 16.92,59.73 16.92,66.91 17.5,67.49 C14.1
N$42
  Top 0.178: R14.2 28.81,67.4 33.68,67.4 34.01,67.07 34.43,67.07 IC1.6
N$43
  Top 0.178: R16.2 23.28,54.69 26.17,54.69 Q5.1
N$44
  Top 0.178: C9.1 39.96,3.67 38.64,3.67 36.65,5.66 Y2.1 36.57,5.74 31.78,10.53 31.78,14.32 U$7.10
N$47
  Top 0.178: R3.1 18.33,5.74 C7.1 18.41,5.74 18.99,5.16 21.63,5.16 | 21.63,5.16 25.1,5.16 25.67,5.74 26.75,5.74 R8.2 | 21.63,5.16 21.63,14.32 U$7.2
N$48
  Top 0.178: LED5.C 19.81,36.03 19.81,33.89 19.9,33.81 R7.2
N$49
  Top 0.2: C1.A 33.71,31.53 30.51,28.31 30.52,24.35 U$7.20
N$50
  Top 0.178: LED8.C 26.17,36.12 26.17,33.89 R6.2
N$51
  Top 0.178: LED6.C 24.44,36.12 24.44,33.81 R4.2
OBD_RX_STATUS/PGC
  Top 0.178: R6.1 27.49,33.81 27.49,29.76 27.9,29.35 27.9,24.39 U$7.22
RESET
  Top 0.178: R1.1 20.8,5.82 20.8,13.91 20.39,14.32 U$7.1
RESET_N
  Top 0.178: R21.2 43.34,43.88 43.34,46.68 42.18,47.84 42.18,62.12 48.62,68.56 J2.10
RST_NVM
  Top 0.178: R5.1 30.63,33.97 30.63,28.93 29.31,27.61 29.31,24.39 U$7.21
RX-STAT
  Top 0.178: R7.1 21.3,33.72 21.3,29.02 25.34,24.97 25.34,24.39 U$7.24
SCL  (via drill 0.5, 0.6)
  Top 0.2: 77.95,53.99 v77.97,54.01 70.78,54.01 JP1.4 70.78,53.35 v71.92,52.21 | v81.52,52.85 85.43,51.02 R41.1 | U3.2 85.45,56.39 v84.93,55.87 | v71.73,49.41 63.17,49.41 JP3.2 60.6,49.39 v60.14,49.85 | v59.58,51.89 U1.16
  Bottom 0.2: v77.97,54.01 78.52,54.01 81.43,52.88 | 81.43,52.88 v81.52,52.85 | v84.93,55.87 84.42,55.87 81.43,52.88 | v71.92,52.21 71.92,49.59 v71.73,49.41 | v60.14,49.85 60.14,51.33 v59.58,51.89
SDA  (via drill 0.6)
  Top 0.2: U3.4 86.27,57.39 | R40.1 87.33,53.64 87.33,53.82 86.99,54.16 86.44,54.16 v86.27,54.22 86.27,54.88 86.31,54.92 U3.4 | U3.4 | U1.17 55.2,52.86 60.86,52.86 61.79,51.93 JP3.3 65.79,51.92 70.4,56.53 JP1.3
  Bottom 0.2: v86.27,54.22 86.47,49.76 81.99,49.74 79.59,49.74 72.8,56.53 JP1.3
SDO_A/G  (via drill 0.6)
  Top 0.2: 86.75,57.58 U3.5 86.76,57.57 86.76,56.27 87.37,55.66 88.76,55.66 89.22,55.2 v89.22,53.15 89.22,53.3 | JP2.1 104.03,50.14 102.37,51.8 | 102.37,51.8 96.37,51.8 v96.29,51.72 | R36.1 97.86,56.31 102.37,51.8
  Bottom 0.2: v96.29,51.72 90.65,51.72 v89.22,53.15
SDO_M  (via drill 0.6 pad 1.02)
  Top 0.2: JP2.2 103.09,52.68 v103.08,52.66 | R38.1 v91.7,54.55 91.32,54.55 89.52,56.35 87.76,56.35 87.31,56.8 87.31,57.55 U3.6
  Bottom 0.2: v103.08,52.66 93.59,52.66 v91.7,54.55
TX-STAT
  Top 0.178: R4.1 23.2,33.72 23.2,28.44 26.67,24.97 26.67,24.39 U$7.23
UART_RX  (via drill 0.38)
  Top 0.178: v53.16,51.22 53.16,52.05 54.98,53.87 55.15,53.87 U1.18 | v41.03,39.09 37.81,39.09 36.74,38.02 36.74,35.46 37.4,34.8 37.4,27.94 34.34,24.89 34.34,24.39 U$7.17 34.34,24.31 34.34,23.73 35.17,22.91 35.99,22.91 36.16,23.07 36.16,25.47 39.54,28.85 39.54,32.98 R9.1
  Bottom 0.178: v41.03,39.09 v53.16,51.22
UART_TX  (via drill 0.38)
  Top 0.178: v52.75,52.63 54.98,54.86 55.15,54.86 U1.19 | v39.46,38.43 38.47,38.43 38.06,38.02 38.06,27.86 35.66,25.47 35.66,24.39 U$7.16
  Bottom 0.178: v52.75,52.63 52.75,51.72 v39.46,38.43

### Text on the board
tNames: GND | GND | GND | GND | 3.3V | DEN A/G | INT2 A/G | RESET_N | JTAG TDI | INT1 A/G | JTAG TDO | JTAG TCKC | JTAG TMSC | INT1 M | GND | DRDY M | BOARD LSM | GND | CS M | SDA | CS A/G | GND | SCL | SDA | SDO_M | SDO_A/G | SCL | BOARD LSM | BUS NEGATIVE | BUS POSITIVE | GND | CAN LOW | CAN HIGH | L LINE | K LINE | +12V | JB's PCB© / Group33 / Sp2017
